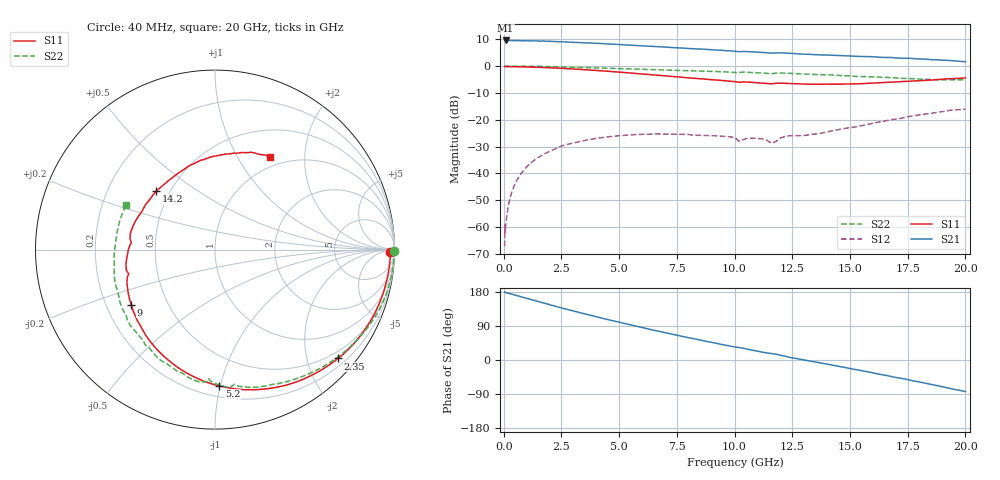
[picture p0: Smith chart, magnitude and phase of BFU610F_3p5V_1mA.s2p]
! Filename:  P:\Prog\Test\Noise\ATS_data\Testdata_Net\SplitFiles\BFU610_2W_A5_HighFreq_3.5V_1mA_D.s2p
! Date/Time: Wed 10/Aug/2011 16:56:21
! BFU610_2W_A5_HighFreq_Bias1_3.5V_1mA_10mA_R.s2p
! MDIF S-parameter v. bias file
! BFU610_2W_A5_HighFreq_3.5V_1mA_10mA
! Date/time Mon Aug 08 14:10:09 2011
! bias mode 1
! bias variable = I_out
! VAR bias_var= 1
! VAR V_out= 3.5010
! VAR I_out= 0.9950
! VAR V_in= 0.8461
! VAR I_in= 0.0071
! Device data file deembeded for feedlines and parallel
! Original file: \SplitFiles\BFU610_2W_A5_HighFreq_3.5V_1mA_R.s2p
! Feed-files: PR003V01_101208_Feed1.s2p, PR003V01_101208_Feed2.s2p
! Parallel-file: PR003V01_101208_Par.s2p
# MHz S MA R 50
!  Freq-MHz  S11-mag  S11-arg  S21-mag  S21-arg  S12-mag  S12-arg  S22-mag  S22-arg
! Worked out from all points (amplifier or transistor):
!   167 points, 40 MHz to 20 GHz, reference 50 ohm
!   highest |S21| = 9.5 dB at 80 MHz (marker M1)
!   |S21| within 3 dB of that: start of sweep to 7.996 GHz
!   unconditionally stable (mu >= 1): 7.93 GHz to end of sweep
!   at 550 MHz: K = -0.02, MSG = 26.2 dB, |S12| = -42.9 dB
!   at 4.2 GHz: K = 0.38, MSG = 17.6 dB, |S12| = -26.7 dB
!   at 20 GHz: K = 1.06, MAG = 7.3 dB, |S12| = -16.0 dB
!   S11 on the Smith chart (normalised r, x): 40 MHz: 67, -37; 2.35 GHz: 0.35, -2.60; 5.2 GHz: 0.28, -0.99; 9 GHz: 0.31, -0.27; 14.2 GHz: 0.42, +0.35; 20 GHz: 0.85, +1.38
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40  0.9773 -0.7  2.999 179.0  0.000443 85.2  0.9978 -0.4
50  0.9708 -1.2  2.986 179.2  0.001108 90.2  0.9981 -0.4
60  0.977 -0.8  2.992 178.3  0.0008023 78.8  0.9985 -0.5
80  0.9772 -1.4  2.999 178.3  0.0009405 90.6  0.9984 -0.7
140  0.9772 -2.5  2.985 177.4  0.001712 91.1  0.9983 -1.3
280  0.9758 -5.0  2.981 175.0  0.003544 90.5  0.9981 -2.7
700  0.9701 -12.5  2.964 167.8  0.009253 84.4  0.9954 -6.7
1350  0.9539 -24.0  2.952 156.7  0.01793 75.2  0.9878 -12.9
2350  0.9153 -41.5  2.856 140.0  0.0308 63.1  0.9678 -22.2
3400  0.8634 -59.1  2.726 123.4  0.04032 49.2  0.9419 -31.4
4300  0.8129 -73.8  2.619 109.8  0.04676 39.4  0.9174 -38.8
5200  0.7599 -88.2  2.49 96.8  0.05126 30.7  0.8921 -45.9
6800  0.6673 -113.2  2.28 74.6  0.05439 17.1  0.8491 -58.1
9000  0.5581 -146.8  2.017 46.7  0.05061 6.7  0.7972 -74.2
10200  0.4993 -164.4  1.853 32.9  0.03971 0.4  0.7581 -81.7
11600  0.4676 175.2  1.742 17.0  0.03636 10.3  0.7202 -92.8
12000  0.4801 168.9  1.763 12.4  0.04602 25.0  0.7431 -96.0
13400  0.4608 146.6  1.637 -4.2  0.05398 23.1  0.6999 -109.8
14200  0.462 134.9  1.594 -13.2  0.06212 26.5  0.6831 -117.8
16800  0.504 99.2  1.445 -43.6  0.1005 19.2  0.6088 -149.5
18400  0.547 79.3  1.331 -63.3  0.1303 7.0  0.565 -175.2
20000  0.6018 59.5  1.204 -83.3  0.1583 -9.6  0.5528 153.4
